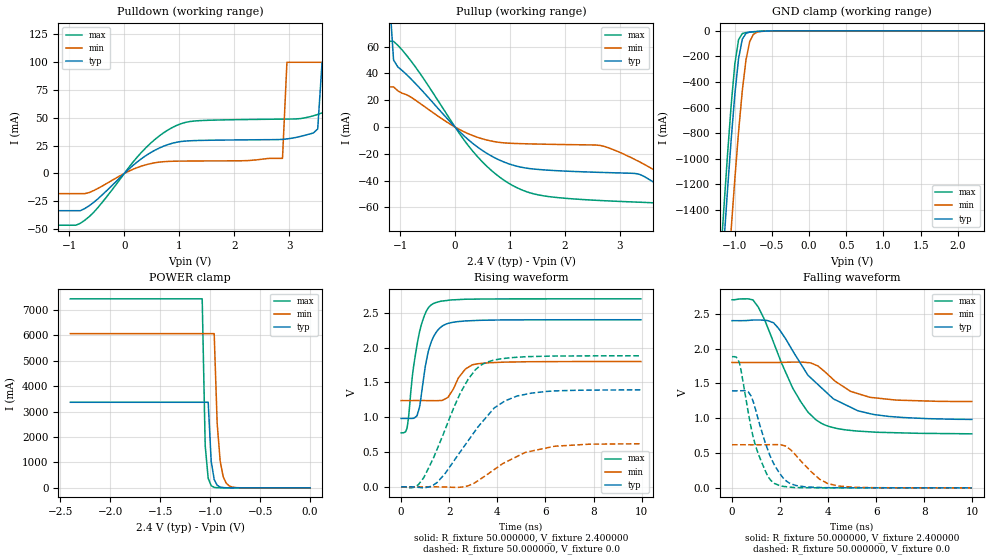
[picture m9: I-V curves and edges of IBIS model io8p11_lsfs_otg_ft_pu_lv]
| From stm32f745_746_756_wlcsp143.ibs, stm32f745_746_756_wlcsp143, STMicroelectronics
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|   Model io8p11_lsfs_otg_ft_pu_lv
[Model]  io8p11_lsfs_otg_ft_pu_lv
Model_type I/O
Polarity   Non-Inverting
Enable   Active-Low
Vinl =   0.720000V
Vinh =   1.680000V
Vmeas =  1.200000V
Cref =   30.000000pF
Rref =   100.000000M
Vref =   0.0V
C_comp   7.971100pF   7.737700pF   8.264100pF
[Temperature Range]   25.000000   0.125000k   -40.000000
[Pullup Reference]   2.400000V   1.800000V   2.700000V
[Pulldown Reference]   0.0V   0.0V   0.0V
[POWER Clamp Reference]   2.400000V   1.800000V   2.700000V
[GND Clamp Reference]   0.0V   0.0V   0.0V
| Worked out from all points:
|   slope of the pulldown table from 0 to 0.36 V, typ, clamps not added: 24.1 ohm
|   slope of the pullup table from 0 to 0.36 V, typ, clamps not added: 26.8 ohm
|   GND clamp passes 1 mA (typ) near -0.52 V on its own axis
|   POWER clamp passes 1 mA (typ) near -0.81 V on its own axis
|   rising waveform, R_fixture 50.000000, V_fixture 2.400000: 20-80 % time 478ps typ, 590ps min, 479ps max; typ from 0.983 V to 2.4 V
|   rising waveform, R_fixture 50.000000, V_fixture 0.0: 20-80 % time 1.82ns typ, 1.82ns min, 1.43ns max; typ from 0.001 V to 1.39 V
|   falling waveform, R_fixture 50.000000, V_fixture 2.400000: 20-80 % time 2.01ns typ, 1.46ns min, 1.54ns max; typ from 2.4 V to 0.983 V
|   falling waveform, R_fixture 50.000000, V_fixture 0.0: 20-80 % time 865ps typ, 1.06ns min, 756ps max; typ from 1.39 V to 0.001 V
[Pulldown]
|Voltage   I(typ)   I(min)   I(max)
-2.4V     -33.44mA   -18.11mA   -46.51mA
-800mV    -33.44mA   -18.11mA   -44.78mA
1.04V     28.81mA    11.14mA    44.91mA
2.88V     30.7mA     13.62mA    48.89mA
2.96V     31.1mA     100mA      48.94mA
3.52V     40mA       100mA      53.06mA
3.6V      100mA      100mA      54.54mA
3.92V     100mA      100mA      60mA
4V        100mA      100mA      100mA
4.4V      100mA      100mA      100mA
4.48V     100mA      100mA      1A
4.8V      100mA      100mA      1A
[Pullup]
|Voltage   I(typ)   I(min)   I(max)
-2.4V     100mA      1A         100mA
-1.6V     100mA      1A         100mA
-1.52V    100mA      30mA       100mA
-1.28V    100mA      30mA       100mA
-1.2V     100mA      30mA       64mA
-1.12V    50mA       30mA       64mA
-1.04V    44.8mA     27mA       60.9mA
320mV     -12.14mA   -6.322mA   -17.91mA
1.12V     -29.18mA   -12.28mA   -45.16mA
3.36V     -35.34mA   -26mA      -56.09mA
4V        -52.4mA    -42mA      -67mA
4.72V     -74mA      -42mA      -94.7mA
[GND_clamp]
|Voltage   I(typ)   I(min)   I(max)
-2.4V     -9.765A    -9.942A    -9.572A
-1.2V     -2.124A    -2.851A    -1.855A
-1.15V    -1.682A    -2.408A    -1.408A
-1.1V     -1.256A    -1.975A    -979.8mA
-1.05V    -854.9mA   -1.556A    -584.5mA
-1V       -496.5mA   -1.158A    -257.5mA
-950mV    -217.7mA   -789.6mA   -69.52mA
-900mV    -65.57mA   -469.8mA   -21.5mA
-850mV    -19.64mA   -226.4mA   -13.56mA
-800mV    -9.753mA   -84.21mA   -10.47mA
-700mV    -4.923mA   -9.884mA   -5.807mA
2.35V     0A         0A         0A
[POWER_clamp]
|Voltage   I(typ)   I(min)   I(max)
-2.4V     3.365A     6.064A     7.43A
-1.08V    3.365A     6.064A     7.43A
-1.05V    3.365A     6.064A     1.669A
-1.02V    3.365A     6.064A     375.2mA
-990mV    1.047A     6.064A     84.45mA
-960mV    325.8mA    6.064A     19.12mA
-930mV    101.4mA    2.529A     4.431mA
-900mV    31.63mA    1.055A     1.12mA
-870mV    9.908mA    440.1mA    365.5uA
-840mV    3.145mA    183.6mA    185.6uA
-720mV    90.15uA    5.596mA    88.88uA
0V        0A         0A         0A
[Ramp]
| variable   typ   min   max
dV/dt_r  0.83451/1.81532n   0.36964/1.81297n   1.12819/1.42946n
dV/dt_f  0.84751/2.01223n   0.33474/1.45875n   1.15296/1.53881n
R_load = 50.000000
[Rising Waveform]
R_fixture= 50.000000
V_fixture= 2.400000
V_fixture_min= 1.800000
V_fixture_max= 2.700000
|time   V(typ)   V(min)   V(max)
0s        982.7mV    1.24V      776.1mV
260.3ps   982.3mV    1.24V      874.2mV
480.5ps   984.3mV    1.24V      1.633V
660.7ps   1.023V     1.24V      2.037V
780.8ps   1.175V     1.24V      2.249V
981ps     1.677V     1.24V      2.471V
1.321ns   2.137V     1.238V     2.629V
1.942ns   2.346V     1.284V     2.679V
2.983ns   2.387V     1.755V     2.696V
9.97ns    2.4V       1.8V       2.7V
[Rising Waveform]
R_fixture= 50.000000
V_fixture= 0.0
V_fixture_min= 0.0
V_fixture_max= 0.0
|time   V(typ)   V(min)   V(max)
0s        869.7uV    836uV      699.2uV
600.6ps   -2.385mV   833.1uV    3.906mV
940.9ps   -10.94mV   852.8uV    133.3mV
1.502ns   64.99mV    716uV      545.8mV
2.462ns   506mV      -4.107mV   1.348V
3.083ns   806.9mV    64mV       1.681V
3.383ns   937.7mV    132.5mV    1.761V
4.304ns   1.232V     348.8mV    1.845V
5.425ns   1.347V     514.4mV    1.872V
9.97ns    1.393V     619.1mV    1.883V
[Falling Waveform]
R_fixture= 50.000000
V_fixture= 2.400000
V_fixture_min= 1.800000
V_fixture_max= 2.700000
|time   V(typ)   V(min)   V(max)
0s        2.4V       1.8V       2.7V
880.9ps   2.409V     1.8V       2.693V
1.361ns   2.405V     1.8V       2.409V
1.722ns   2.37V      1.8V       2.094V
2.503ns   1.981V     1.805V     1.449V
2.843ns   1.791V     1.805V     1.246V
3.724ns   1.435V     1.707V     925.4mV
4.925ns   1.158V     1.386V     825.2mV
5.726ns   1.067V     1.301V     804.8mV
9.97ns    982.7mV    1.24V      776.1mV
[Falling Waveform]
R_fixture= 50.000000
V_fixture= 0.0
V_fixture_min= 0.0
V_fixture_max= 0.0
|time   V(typ)   V(min)   V(max)
0s        1.393V     619.1mV    1.883V
320.3ps   1.394V     619.1mV    1.78V
780.8ps   1.326V     619mV      889.1mV
981ps     1.122V     618.9mV    603.3mV
1.221ns   830.2mV    618.9mV    378.9mV
1.762ns   332.7mV    621.6mV    64.22mV
2.482ns   54.53mV    531.2mV    8.707mV
3.644ns   5.959mV    124.8mV    1.17mV
4.424ns   2.454mV    27.15mV    1.155mV
9.97ns    869.7uV    836uV      699.2uV
